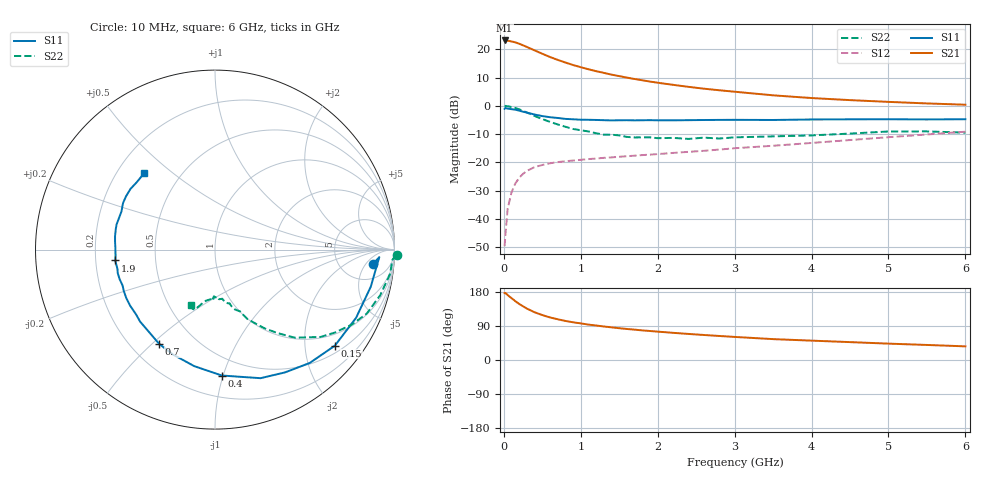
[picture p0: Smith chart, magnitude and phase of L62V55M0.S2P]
!  INFINEON TECHNOLOGIES Small Signal Semiconductors
! BFR380L3 , Si-NPN RF-Transistor in TSLP-3-1
!  Vce=2.5 V,  Ic=5 mA
! Common Emitter S-Parameters:  07. March 2005
#  GHz  S  MA  R  50
! f  S11  S21  S12  S22
! GHz  Mag  Ang  Mag  Ang  Mag  Ang  Mag  Ang
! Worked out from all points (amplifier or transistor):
!   36 points, 10 MHz to 6 GHz, reference 50 ohm
!   highest |S21| = 23.1 dB at 10 MHz (marker M1)
!   |S21| within 3 dB of that: start of sweep to 357.4 MHz
!   unconditionally stable (mu >= 1): 2.359 GHz to 4.732 GHz
!   at 250 MHz: K = 0.16, MSG = 22.7 dB, |S12| = -24.0 dB
!   at 1.4 GHz: K = 0.77, MSG = 14.6 dB, |S12| = -18.2 dB
!   at 6 GHz: K = 0.94, MSG = 4.8 dB, |S12| = -9.1 dB
!   S11 on the Smith chart (normalised r, x): 10 MHz: 11, -8; 150 MHz: 0.67, -2.70; 400 MHz: 0.36, -0.99; 700 MHz: 0.31, -0.53; 1.9 GHz: 0.28, -0.05; 6 GHz: 0.31, +0.40
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0.01  0.8849 -5.1  14.34 176.6  0.0033 87.7  1.012 -1.6
0.02  0.9165 -2.6  14.31 176.9  0.0052 90.8  0.9899 -3.3
0.05  0.8922 -13.4  14.2 171.3  0.0152 83.5  0.9849 -7.9
0.1  0.8731 -25.8  13.78 163.2  0.0296 77.2  0.9547 -15.5
0.15  0.8559 -38.7  13.26 155.2  0.0426 70.7  0.9174 -22.9
0.2  0.8231 -50.1  12.55 147.8  0.0534 65.3  0.8685 -28.8
0.25  0.7876 -60.3  11.77 141.7  0.0628 60.6  0.812 -34.7
0.3  0.76 -70.5  10.99 135.6  0.0709 56.4  0.7634 -39.6
0.4  0.7026 -86.9  9.579 125.9  0.0826 50.1  0.6626 -47.8
0.5  0.6595 -100.1  8.345 118.6  0.09 46.6  0.5833 -53.0
0.6  0.6299 -111.8  7.314 112.3  0.0966 43.6  0.5212 -57.6
0.7  0.6107 -120.6  6.502 107.5  0.1012 42.0  0.4695 -61.3
0.9  0.5789 -136.1  5.276 99.5  0.1078 40.7  0.3898 -67.0
1.1  0.5668 -146.5  4.437 93.4  0.1144 41.0  0.3527 -71.4
1.4  0.5524 -158.8  3.566 86.2  0.1225 42.1  0.3085 -76.1
1.9  0.5586 -173.8  2.689 76.5  0.1372 45.8  0.2774 -85.5
2.2  0.5548 179.6  2.354 71.7  0.1471 48.3  0.2713 -87.1
2.8  0.5645 168.2  1.888 63.4  0.1686 52.9  0.2646 -94.8
3.5  0.5627 157.9  1.536 55.1  0.197 55.9  0.2887 -99.9
4.5  0.5779 149.2  1.263 47.2  0.2486 60.0  0.3234 -105.3
5.5  0.5752 139.2  1.104 39.7  0.312 60.4  0.3535 -110.6
6  0.5804 133.0  1.048 36.0  0.3489 59.3  0.3358 -113.4
